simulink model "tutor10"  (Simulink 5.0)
settings: Solver=ode45  SolverMode=SingleTasking  StartTime=0.0  StopTime=10  RelTol=1e-3  AbsTol=1e-3
libraries: simulink x1

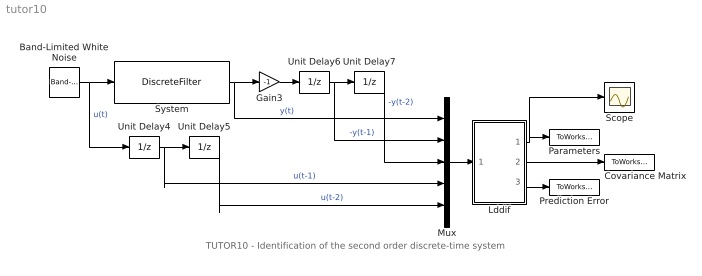
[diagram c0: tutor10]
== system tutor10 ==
  note: TUTOR10 - Identification of the second order discrete-time system
  Band-Limited White Noise : simulink/Sources/Band-Limited White Noise  Cov=[0.1]  Ts=0.1  seed=[23341]
  Covariance Matrix : ToWorkspace  VariableName=CovMatrix  SaveFormat=Array
  Gain3 : Gain  Gain=-1
  Lddif : Subsystem  mask(LDDIF){par=[4,1], L=[0.985], d=[0.01], poc=[0 0 0 0], kov=[10e6], ts=[1]}
      mask prompts: par "No. of estimated parameters and outputs - [n,m]:"; L "Exponential forgetting - [L]:"; d "Bittanti's correction - [d]:"; poc "Initial parameter estimates - [theta(1) ... theta(n)]:"; kov "Covariance matrix (see help, standard - [10e6]):"; ts "Sampling period - [ts]:"
      mask help: LDDIF: + Bittanti's corrections Authors: Lubos Cirka and Miroslav Fikar 1998 - 2006
      mask init:
      | n=par(1); m=par(2);
  Mux : Mux  Inputs=5
  Parameters : ToWorkspace  VariableName=BA  SaveFormat=Array
  Prediction Error : ToWorkspace  VariableName=PredError  SaveFormat=Array
  Scope : Scope
  System : DiscreteFilter  Numerator=[0 0.8 0.2]  Denominator=[1 -0.5 0.06]
  Unit Delay{4..7} (4 alike) : UnitDelay
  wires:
  System/1 -> Mux/1, Gain3/1  "y(t)"
  Unit Delay6/1 -> Mux/2, Unit Delay7/1  "-y(t-1)"
  Gain3/1 -> Unit Delay6/1
  Unit Delay4/1 -> Mux/4, Unit Delay5/1  "u(t-1)"
  Band-Limited White Noise/1 -> Unit Delay4/1, System/1  "u(t)"
  Mux/1 -> Lddif/1("y, z")
  Unit Delay7/1 -> Mux/3  "-y(t-2)"
  Unit Delay5/1 -> Mux/5  "u(t-2)"
  Lddif/2(covariance matrix) -> Covariance Matrix/1
  Lddif/3(prediction error) -> Prediction Error/1
  Lddif/1(theta) -> Parameters/1, Scope/1

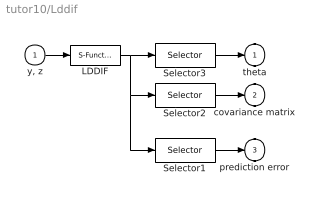
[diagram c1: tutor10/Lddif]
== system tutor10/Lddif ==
  "y, z" : Inport
  LDDIF : S-Function  FunctionName=lddif_s  Parameters=m, n, L, d, poc, kov, ts
  Selector1 : Selector  Elements=[n*m+n*n+1:1:n*m+n*n+m]  InputPortWidth=n*m+n*n+m
  Selector2 : Selector  Elements=[n*m+1:1:n*m+n*n]  InputPortWidth=n*m+n*n+m
  Selector3 : Selector  Elements=[1:1:n*m]  InputPortWidth=n*m+n*n+m
  theta : Outport  InitialOutput=0
  covariance matrix : Outport  Port=2  InitialOutput=0
  prediction error : Outport  Port=3  InitialOutput=0
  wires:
  "y, z"/1 -> LDDIF/1
  LDDIF/1 -> Selector1/1, Selector2/1, Selector3/1
  Selector2/1 -> covariance matrix/1
  Selector3/1 -> theta/1
  Selector1/1 -> prediction error/1
